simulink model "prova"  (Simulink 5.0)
settings: Solver=ode45  StartTime=0.0  StopTime=10.0  RelTol=1e-3
undefined symbols (not defined in the file or in its folder): changeError, sigbuilder_block
libraries: fuzblock x5

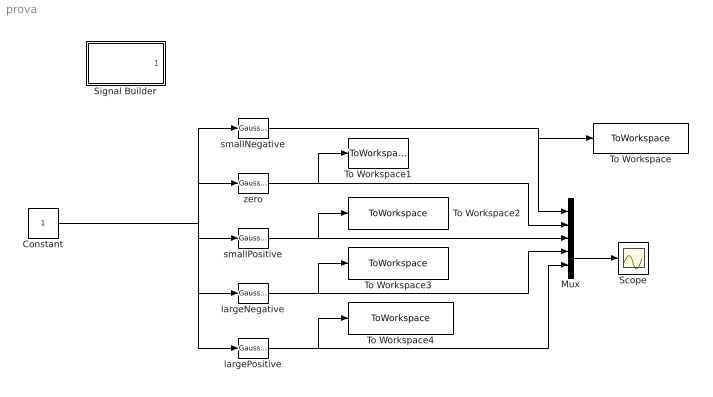
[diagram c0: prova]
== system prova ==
  Constant : Constant
  Mux : Mux  Inputs=5
  Scope : Scope
  Signal Builder : Subsystem  Tag=STV Subsys  StartFcn=sigbuilder_block('start');  StopFcn=sigbuilder_block('stop');  ClipboardFcn=sigbuilder_block('clipboard');
  To Workspace : ToWorkspace  VariableName=small_negative  SampleTime=1/20  SaveFormat=Array
  To Workspace1 : ToWorkspace  VariableName=zero  SampleTime=1/20  SaveFormat=Array
  To Workspace2 : ToWorkspace  VariableName=small_positive  SampleTime=1/20  SaveFormat=Array
  To Workspace3 : ToWorkspace  VariableName=large_negative  SampleTime=1/20  SaveFormat=Array
  To Workspace4 : ToWorkspace  VariableName=large_positive  SampleTime=1/20  SaveFormat=Array
  largeNegative : fuzblock/Membership  Functions/Gaussian MF  sigma=changeError.input(1).mf(4).params(1)  mu=changeError.input(1).mf(4).params(2)
  largePositive : fuzblock/Membership  Functions/Gaussian MF  sigma=changeError.input(1).mf(5).params(1)  mu=changeError.input(1).mf(5).params(2)
  smallNegative : fuzblock/Membership  Functions/Gaussian MF  sigma=changeError.input(1).mf(1).params(1)  mu=changeError.input(1).mf(1).params(2)
  smallPositive : fuzblock/Membership  Functions/Gaussian MF  sigma=changeError.input(1).mf(3).params(1)  mu=changeError.input(1).mf(3).params(2)
  zero : fuzblock/Membership  Functions/Gaussian MF  sigma=changeError.input(1).mf(2).params(1)  mu=changeError.input(1).mf(2).params(2)
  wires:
  Constant/1 -> smallNegative/1, zero/1, smallPositive/1, largeNegative/1, largePositive/1
  smallNegative/1 -> Mux/1, To Workspace/1
  zero/1 -> Mux/2, To Workspace1/1
  smallPositive/1 -> Mux/3, To Workspace2/1
  largeNegative/1 -> Mux/4, To Workspace3/1
  Mux/1 -> Scope/1
  largePositive/1 -> To Workspace4/1, Mux/5

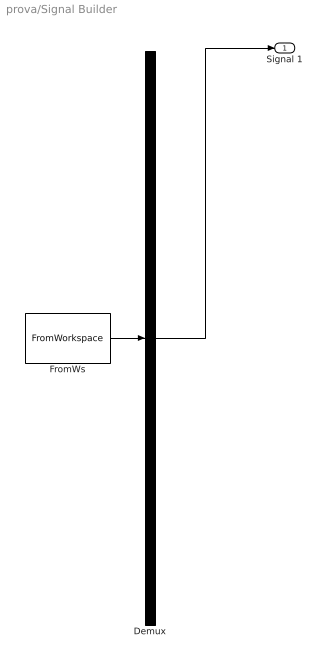
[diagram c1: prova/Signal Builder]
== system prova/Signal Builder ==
  Demux : Demux  Tag=STV Demux  Outputs=1
  FromWs : FromWorkspace  Tag=STV FromWs  VariableName=tuvar  SampleTime=0  SigBuilderData=DataTag0
  Signal 1 : Outport  Tag=STV Outport
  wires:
  Demux/1 -> Signal 1/1
  FromWs/1 -> Demux/1
